| IBIS file stm32l4r9_s9_wlcsp144.ibs
[IBIS ver]   4.2
[File name]   stm32l4r9_s9_wlcsp144.ibs
[File Rev]   1.0
[Date]   01-6-2017
[Source]   Data Created at STMicroelectronics
[Notes]   File originated from ELDO simulations.
[Disclaimer]  This information is for modeling purpose only and is
   not guaranted.
   The information is subject to change without notice.
[Copyright]   Copyright 2017 STMicroelectronics Inc.
|   Component stm32l4r9_s9_wlcsp144
[Component] stm32l4r9_s9_wlcsp144
[Manufacturer] STMicroelectronics
[Package]
| variable   typ   min   max
R_pkg   0.0   0.0   0.0
L_pkg   0.0H   0.0H   0.0H
C_pkg   0.0F   0.0F   0.0F
[Pin]  signal_name   model_name   R_pin   L_pin   C_pin
A1 VSS gnd
A10 PE0 io8prog2m25m50m120m_sudq_ft
A11 PE1 io8prog2m25m50m120m_sudq_ft
A12 VSS gnd
A2 PA14 io8prog2m25m50m120m_sudq_ft
A3 PA15 io8prog2m25m50m120m_sudq_ft
A4 PD0 io8prog2m25m50m120m_sudq_ft
A5 PD5 io8prog2m25m50m120m_sudq_ft
A6 VDD power
A7 PG12 io8prog2m25m50m120m_sudq_ft
A8 VDDIO2 power
A9 PB7 io8prog2m25m50m120m_sudq_i2c_ft
B1 VDD power
B10 PB9 io8prog2m25m50m120m_sudq_i2c_ft
B11 PE2 io8prog2m25m50m120m_sudq_ft
B12 VDD power
B2 VDDUSB power
B3 PA13 io8prog2m25m50m120m_sudq_ft
B4 PC12 io8prog2m25m50m120m_sudq_ft
B5 PD2 io8prog2m25m50m120m_sudq_ft
B6 VSS power
B7 PG10 io8prog2m25m50m120m_sudq_ft
B8 PB3 io8prog2m25m50m120m_sudq_ft
B9 PH3-BOOT0 io8prog2m25m50m120m_sudq_ft
C1 PA11 io8usblsfs_otg2
C10 PB8 io8prog2m25m50m120m_sudq_i2c_ft
C11 PE3 io8prog2m25m50m120m_sudq_ft
C12 PE4 io8prog2m25m50m120m_sudq_ft
C2 PA12 io8usblsfs_otg2
C3 PC10 io8prog2m25m50m120m_sudq_ft
C4 PC11 io8prog2m25m50m120m_sudq_ft
C5 PD1 io8prog2m25m50m120m_sudq_ft
C6 PD4 io8prog2m25m50m120m_sudq_ft
C7 PG9 io8prog2m25m50m120m_sudq_ft
C8 PB4 io8prog2m25m50m120m_sudq_i2c_ft
C9 PB6 io8prog2m25m50m120m_sudq_i2c_ft
D1 PC8 io8prog2m25m50m120m_sudq_ft
D10 PE6 io8prog2m25m50m120m_sudq_ft
D11 PC13 io8prog2m25m50m120m_sudq_ft
D12 VSS power
D2 PC9 io8prog2m25m50m120m_sudq_ft
D3 PA8 io8prog2m25m50m120m_sudq_ft
D4 PA9 power
D5 PA10 io8usb_id_otg20_lcd4_ft_ms
D6 PD3 io8prog2m25m50m120m_sudq_ft
D7 PD7 io8prog2m25m50m120m_sudq_ft
D8 PG13 io8prog2m25m50m120m_sudq_i2c_ft
D9 PE5 io8prog2m25m50m120m_sudq_ft
E1 PG7 io8prog2m25m50m120m_sudq_i2c_ft
E10 VBAT power
E11 PC14-OSC32_IN io8prog2m25m50m120m_sudq_ft
E12 PC15-OSC32_OUT io8prog2m25m50m120m_sudq_ft
E2 PG8 io8prog2m25m50m120m_sudq_i2c_ft
E3 VDDIO2 power
E4 PC6 io8prog2m25m50m120m_sudq_ft
E5 PG6 io8prog2m25m50m120m_sudq_ft
E6 PC7 io8prog2m25m50m120m_sudq_ft
E7 PD6 io8prog2m25m50m120m_sudq_ft
E8 PB5 io8prog2m25m50m120m_sudq_ft
E9 PF0 io8prog2m25m50m120m_sudq_i2c_ft
F1 PD15 io8prog2m25m50m120m_sudq_ft
F10 PF4 io8prog2m25m50m120m_sudq_ft
F11 PF3 io8prog2m25m50m120m_sudq_ft
F12 PF2 io8prog2m25m50m120m_sudq_ft
F2 PG2 io8prog2m25m50m120m_sudq_ft
F3 PD14 io8prog2m25m50m120m_sudq_ft
F4 PD12 io8prog2m25m50m120m_sudq_ft
F5 PG3 io8prog2m25m50m120m_sudq_ft
F6 PG4 io8prog2m25m50m120m_sudq_ft
F7 PG5 io8prog2m25m50m120m_sudq_ft
F8 PF1 io8prog2m25m50m120m_sudq_i2c_ft
F9 PF5 io8prog2m25m50m120m_sudq_ft
G1 VSS gnd
G10 PF6 io8prog2m25m50m120m_sudq_ft
G11 VSS gnd
G12 VDD power
G2 VDD power
G3 PD13 io8prog2m25m50m120m_sudq_ft
G4 PD11 io8prog2m25m50m120m_sudq_ft
G5 PD10 io8prog2m25m50m120m_sudq_ft
G6 PE9 io8prog2m25m50m120m_sudq_ft
G7 PF14 io8prog2m25m50m120m_sudq_i2c_ft
G8 PA5 io8prog2m25m50m120m_sudq_ft
G9 PF7 io8prog2m25m50m120m_sudq_ft
H1 PD9 io8prog2m25m50m120m_sudq_ft
H10 PF10 io8prog2m25m50m120m_sudq_ft
H11 NRST ioreset_ft_v33
H12 PH0-OSC_IN io8prog2m25m50m120m_sudq_ft
H2 PD8 io8prog2m25m50m120m_sudq_ft
H3 PB14 io8prog2m25m50m120m_sudq_i2c_ft
H4 PB13 io8prog2m25m50m120m_sudq_i2c_ft
H5 PE14 io8prog2m25m50m120m_sudq_ft
H6 PE8 io8prog2m25m50m120m_sudq_ft
H7 PB1 io8prog2m25m50m120m_sudq_ft
H8 PA2 io8prog2m25m50m120m_sudq_ft
H9 PC2 io8prog2m25m50m120m_sudq_ft
J1 DSI_D1N NC
J10 PC3 io8prog2m25m50m120m_sudq_ft
J11 PC0 io8prog2m25m50m120m_sudq_i2c_ft
J12 PH1-OSC_OUT io8prog2m25m50m120m_sudq_ft
J2 DSI_D1P NC
J3 PB15 io8prog2m25m50m120m_sudq_ft
J4 PB12 io8prog2m25m50m120m_sudq_ft
J5 PE13 io8prog2m25m50m120m_sudq_ft
J6 PF15 io8prog2m25m50m120m_sudq_i2c_ft
J7 PB2 io8prog2m25m50m120m_sudq_ft
J8 PA6 io8prog2m25m50m120m_sudq_ft
J9 PA0 io8prog2m25m50m120m_sudq_ft
K1 DSI_CKP NC
K10 PA1 io8prog2m25m50m120m_sudq_ft
K11 VSSA/VREF- gnd
K12 PC1 io8prog2m25m50m120m_sudq_i2c_ft
K2 DSI_CKN NC
K3 VSSDSI gnd
K4 PE15 io8prog2m25m50m120m_sudq_ft
K5 PE10 io8prog2m25m50m120m_sudq_ft
K6 PG0 io8prog2m25m50m120m_sudq_ft
K7 PF11 io8prog2m25m50m120m_sudq_ft
K8 PC5 io8prog2m25m50m120m_sudq_ft
K9 PA4 io8prog2m25m50m120m_sudq_ft
L1 DSI_D0P NC
L10 PA3 io8prog2m25m50m120m_sudq_ft
L11 VREF+ power
L12 VDDA power
L2 DSI_D0N NC
L3 VCAPDSI NC
L4 PB10 io8prog2m25m50m120m_sudq_i2c_ft
L5 PE11 io8prog2m25m50m120m_sudq_ft
L6 PG1 io8prog2m25m50m120m_sudq_ft
L7 VDD power
L8 PF12 io8prog2m25m50m120m_sudq_ft
L9 PC4 io8prog2m25m50m120m_sudq_ft
M1 VDD power
M10 PA7 io8prog2m25m50m120m_sudq_i2c_ft
M11 VDD power
M12 VSS gnd
M2 VDD power
M3 VSS gnd
M4 PB11 io8prog2m25m50m120m_sudq_i2c_ft
M5 PE12 io8prog2m25m50m120m_sudq_ft
M6 PE7 io8prog2m25m50m120m_sudq_ft
M7 PF13 io8prog2m25m50m120m_sudq_ft
M8 VSS gnd
M9 PB0 io8prog2m25m50m120m_sudq_ft
[Diff Pin]   inv_pin   vdiff   tdelay_typ  tdelay_min  tdelay_max
C1 C2 200mV   NA   NA   NA
[Model Selector] io8prog2m25m50m120m_sudq_ft
io8p00_sudq_ft_pd_lv  "SPEED00, PD=40kOhm - 1P8V"
io8p00_sudq_ft_pu_lv  "SPEED00, PU=40kOhm - 1P8V"
io8p00_sudq_ft_lv  "SPEED00 - 1P8V"
io8p00_sudq_ft_pd  "SPEED00, PD=40kOhm - 3P3V"
io8p00_sudq_ft_pu  "SPEED00, PU=40kOhm - 3P3V"
io8p00_sudq_ft  "SPEED00 - 3P3V"
io8p01_sudq_ft_pd_lv  "SPEED01, PD=40kOhm - 1P8V"
io8p01_sudq_ft_pu_lv  "SPEED01, PU=40kOhm - 1P8V"
io8p01_sudq_ft_lv  "SPEED01 - 1P8V"
io8p01_sudq_ft_pd  "SPEED01, PD=40kOhm - 3P3V"
io8p01_sudq_ft_pu  "SPEED01, PU=40kOhm - 3P3V"
io8p01_sudq_ft  "SPEED01 - 3P3V"
io8p10_sudq_ft_pd_lv  "SPEED10, PD=40kOhm - 1P8V"
io8p10_sudq_ft_pu_lv  "SPEED10, PU=40kOhm - 1P8V"
io8p10_sudq_ft_lv  "SPEED10 - 1P8V"
io8p10_sudq_ft_pd  "SPEED10, PD=40kOhm - 3P3V"
io8p10_sudq_ft_pu  "SPEED10, PU=40kOhm - 3P3V"
io8p10_sudq_ft  "SPEED10 - 3P3V"
io8p11_sudq_ft_pd_lv  "SPEED11, PD=40kOhm - 1P8V"
io8p11_sudq_ft_pu_lv  "SPEED11, PU=40kOhm - 1P8V"
io8p11_sudq_ft_lv  "SPEED11 - 1P8V"
io8p11_sudq_ft_pd  "SPEED11, PD=40kOhm - 3P3V"
io8p11_sudq_ft_pu  "SPEED11, PU=40kOhm - 3P3V"
io8p11_sudq_ft  "SPEED11 - 3P3V"
[Model Selector] io8prog2m25m50m120m_sudq_i2c_ft
io8prog_1v8_i2c_pd  "5V Tol GPIO 1.8V range i2c functionality with pull down"
io8prog_1v8_i2c_pu  "5V Tol GPIO 1.8V range i2c functionality with pull up"
io8prog_1v8_i2c  "5V Tol GPIO 1.8V range i2c functionality"
io8prog_3v3_i2c_pd  "5V Tol GPIO 3.3V range i2c functionality with pull down"
io8prog_3v3_i2c_pu  "5V Tol GPIO 3.3V range i2c functionality with pull up"
io8prog_3v3_i2c  "5V Tol GPIO 3.3V range i2c functionality"
io8prog_1v8_pd_00  "5V Tol GPIO 1.8V range with pd speed 00"
io8prog_1v8_pu_00  "5V Tol GPIO 1.8V range with pu speed 00"
io8prog_1v8_00  "5V Tol GPIO 1.8V range speed 00"
io8prog_3v3_pd_00  "5V Tol GPIO 3.3V range with pd speed 00"
io8prog_3v3_pu_00  "5V Tol GPIO 3.3V range with pu speed 00"
io8prog_3v3_00  "5V Tol GPIO 3.3V range speed 00"
io8prog_1v8_pd_01  "5V Tol GPIO 1.8V range with pd speed 01"
io8prog_1v8_pu_01  "5V Tol GPIO 1.8V range with pu speed 01"
io8prog_1v8_01  "5V Tol GPIO 1.8V range speed 01"
io8prog_3v3_pd_01  "5V Tol GPIO 3.3V range with pd speed 01"
io8prog_3v3_pu_01  "5V Tol GPIO 3.3V range with pu speed 01"
io8prog_3v3_01  "5V Tol GPIO 3.3V range speed 01"
io8prog_1v8_pd_10  "5V Tol GPIO 1.8V range with pd speed 10"
io8prog_1v8_pu_10  "5V Tol GPIO 1.8V range with pu speed 10"
io8prog_1v8_10  "5V Tol GPIO 1.8V range speed 10"
io8prog_3v3_pd_10  "5V Tol GPIO 3.3V range with pd speed 10"
io8prog_3v3_pu_10  "5V Tol GPIO 3.3V range with pu speed 10"
io8prog_3v3_10  "5V Tol GPIO 3.3V range speed 10"
io8prog_1v8_pd_11  "5V Tol GPIO 1.8V range with pd speed 11"
io8prog_1v8_pu_11  "5V Tol GPIO 1.8V range with pu speed 11"
io8prog_1v8_11  "5V Tol GPIO 1.8V range speed 11"
io8prog_3v3_pd_11  "5V Tol GPIO 3.3V range with pd speed 11"
io8prog_3v3_pu_11  "5V Tol GPIO 3.3V range with pu speed 11"
io8prog_3v3_11  "5V Tol GPIO 3.3V range speed 11"
[Model Selector] io8usb_id_otg20_lcd4_ft_ms
io8usbid_1v8_id_pu  "ID 1V8 range with pull up"
io8usbid_3v3_id_pu  "ID 3V3 range with pull up"
io8usbid_1v8_id  "ID 1V8 range"
io8usbid_3v3_id  "ID 3V3 range"
io8usbid_1v8_pd_00  "GPIO 1.8V range with pd speed 00"
io8usbid_1v8_pu_00  "GPIO 1.8V range with pu speed 00"
io8usbid_1v8_00  "GPIO 1.8V range speed 00"
io8usbid_3v3_pd_00  "GPIO 3.3V range with pd speed 00"
io8usbid_3v3_pu_00  "GPIO 3.3V range with pu speed 00"
io8usbid_3v3_00  "GPIO 3.3V range speed 00"
io8usbid_1v8_pd_01  "GPIO 1.8V range with pd speed 01"
io8usbid_1v8_pu_01  "GPIO 1.8V range with pu speed 01"
io8usbid_1v8_01  "GPIO 1.8V range speed 01"
io8usbid_3v3_pd_01  "GPIO 3.3V range with pd speed 01"
io8usbid_3v3_pu_01  "GPIO 3.3V range with pu speed 01"
io8usbid_3v3_01  "GPIO 3.3V range speed 01"
io8usbid_1v8_pd_10  "GPIO 1.8V range with pd speed 10"
io8usbid_1v8_pu_10  "GPIO 1.8V range with pu speed 10"
io8usbid_1v8_10  "GPIO 1.8V range speed 10"
io8usbid_3v3_pd_10  "GPIO 3.3V range with pd speed 10"
io8usbid_3v3_pu_10  "GPIO 3.3V range with pu speed 10"
io8usbid_3v3_10  "GPIO 3.3V range speed 10"
io8usbid_1v8_pd_11  "GPIO 1.8V range with pd speed 11"
io8usbid_1v8_pu_11  "GPIO 1.8V range with pu speed 11"
io8usbid_1v8_11  "GPIO 1.8V range speed 11"
io8usbid_3v3_pd_11  "GPIO 3.3V range with pd speed 11"
io8usbid_3v3_pu_11  "GPIO 3.3V range with pu speed 11"
io8usbid_3v3_11  "GPIO 3.3V range speed 11"
[Model Selector] io8usblsfs_otg2
usb_ls_pd  "USB Low Speed mode - Pull Down"
usb_ls_pu2  "USB Low Speed mode - Pull up 2"
usb_ls_pu  "USB Low Speed mode - Pull up"
usb_fs  "USB Low Speed mode"
usb_fs_pd  "USB Full Speed mode - Pull Down"
usb_fs_pu2  "USB Full Speed mode - Pull up 2"
usb_fs_pu  "USB Full Speed mode - Pull up"
[Model Selector] ioreset_ft_v33
ioreset_1v2_pu  "RESET 1.2V range with PU"
ioreset_1v2  "RESET 1.2V range"
ioreset_1v8_pu  "RESET 1.8V range with PU"
ioreset_1v8  "RESET 1.8V range"
ioreset_3v3_pu  "RESET 3.3V range with PU"
ioreset_3v3  "RESET 3.3V range"
| Models and submodels in the file (95): io8p00_sudq_ft_pd_lv (I/O), io8p00_sudq_ft_pu_lv (I/O), io8p00_sudq_ft_lv (I/O), io8p00_sudq_ft_pd (I/O), io8p00_sudq_ft_pu (I/O), io8p00_sudq_ft (I/O), io8p01_sudq_ft_pd_lv (I/O), io8p01_sudq_ft_pu_lv (I/O), io8p01_sudq_ft_lv (I/O), io8p01_sudq_ft_pd (I/O), io8p01_sudq_ft_pu (I/O), io8p01_sudq_ft (I/O), io8p10_sudq_ft_pd_lv (I/O), io8p10_sudq_ft_pu_lv (I/O), io8p10_sudq_ft_lv (I/O), io8p10_sudq_ft_pd (I/O), io8p10_sudq_ft_pu (I/O), io8p10_sudq_ft (I/O), io8p11_sudq_ft_pd_lv (I/O), io8p11_sudq_ft_pu_lv (I/O), io8p11_sudq_ft_lv (I/O), io8p11_sudq_ft_pd (I/O), io8p11_sudq_ft_pu (I/O), io8p11_sudq_ft (I/O), io8prog_1v8_i2c_pd (I/O), io8prog_1v8_i2c_pu (I/O), io8prog_1v8_i2c (I/O), io8prog_3v3_i2c_pd (I/O), io8prog_3v3_i2c_pu (I/O), io8prog_3v3_i2c (I/O), io8prog_1v8_pd_00 (I/O), io8prog_1v8_pu_00 (I/O), io8prog_1v8_00 (I/O), io8prog_3v3_pd_00 (I/O), io8prog_3v3_pu_00 (I/O), io8prog_3v3_00 (I/O), io8prog_1v8_pd_01 (I/O), io8prog_1v8_pu_01 (I/O), io8prog_1v8_01 (I/O), io8prog_3v3_pd_01 (I/O), io8prog_3v3_pu_01 (I/O), io8prog_3v3_01 (I/O), io8prog_1v8_pd_10 (I/O), io8prog_1v8_pu_10 (I/O), io8prog_1v8_10 (I/O), io8prog_3v3_pd_10 (I/O), io8prog_3v3_pu_10 (I/O), io8prog_3v3_10 (I/O), io8prog_1v8_pd_11 (I/O), io8prog_1v8_pu_11 (I/O), io8prog_1v8_11 (I/O), io8prog_3v3_pd_11 (I/O), io8prog_3v3_pu_11 (I/O), io8prog_3v3_11 (I/O), io8usbid_1v8_id_pu (Input), io8usbid_3v3_id_pu (Input), io8usbid_1v8_id (Input), io8usbid_3v3_id (Input), io8usbid_1v8_pd_00 (I/O), io8usbid_1v8_pu_00 (I/O), io8usbid_1v8_00 (I/O), io8usbid_3v3_pd_00 (I/O), io8usbid_3v3_pu_00 (I/O), io8usbid_3v3_00 (I/O), io8usbid_1v8_pd_01 (I/O), io8usbid_1v8_pu_01 (I/O), io8usbid_1v8_01 (I/O), io8usbid_3v3_pd_01 (I/O), io8usbid_3v3_pu_01 (I/O), io8usbid_3v3_01 (I/O), io8usbid_1v8_pd_10 (I/O), io8usbid_1v8_pu_10 (I/O), io8usbid_1v8_10 (I/O), io8usbid_3v3_pd_10 (I/O), io8usbid_3v3_pu_10 (I/O), io8usbid_3v3_10 (I/O), io8usbid_1v8_pd_11 (I/O), io8usbid_1v8_pu_11 (I/O), io8usbid_1v8_11 (I/O), io8usbid_3v3_pd_11 (I/O)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
